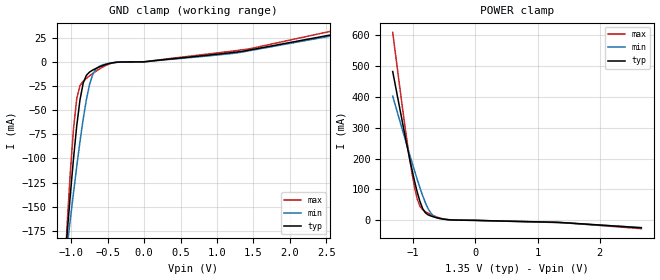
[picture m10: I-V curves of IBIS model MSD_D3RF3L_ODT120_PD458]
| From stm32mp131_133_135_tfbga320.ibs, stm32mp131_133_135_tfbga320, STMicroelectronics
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[Model] MSD_D3RF3L_ODT120_PD458
Model_type   Input
C_comp 2.350pF   2.272pF   2.440pF
Vinh = 810.000mV
Vinl = 540.000mV
[Receiver Thresholds]
Vth   =  0.675V
Vth_min  =  0.6615V
Vth_max  =  0.6885V
Vinh_ac  =  0.160V
Vinh_dc  =  0.090V
Vinl_ac  = -0.160V
Vinl_dc  = -0.090V
Tslew_ac =  5.000ns |Not specified, so set to high value
[Temperature Range]   25.000   125.000   -40.000
[Voltage Range]   1.350V   1.283V   1.450V
[GND Clamp Reference]   0.00V   0.00V   0.00V
[POWER Clamp Reference]   1.350V   1.283V   1.450V
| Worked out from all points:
|   GND clamp passes 1 mA (typ) near -0.43 V on its own axis
|   POWER clamp passes 1 mA (typ) near -0.32 V on its own axis
[GND Clamp]
-1.318V   -446.4mA   -371.4mA   -564.9mA
-1.098V   -221.3mA   -221.2mA   -229.7mA
-1.055V   -178.6mA   -191.9mA   -169mA
-1.011V   -137.8mA   -163.3mA   -114.4mA
-966.7mV  -99.79mA   -135.3mA   -69.1mA
-922.7mV  -66.28mA   -108.3mA   -38.22mA
-834.9mV  -22.17mA   -59.48mA   -20.04mA
-747mV    -10.58mA   -23.42mA   -14.51mA
-659.1mV  -6.847mA   -7.337mA   -9.707mA
-483.3mV  -1.839mA   -1.559mA   -2.399mA
1.45V     12.26mA    11.56mA    13.54mA
2.68V     29.53mA    28.4mA     33.61mA
[Power Clamp]
-1.33V    481.4mA    401.8mA    608.1mA
-1.155V   297.6mA    279.3mA    336.2mA
-1.023V   166.5mA    189.5mA    156.2mA
-978.8mV  126.8mA    160.4mA    107mA
-934.9mV  90.92mA    132mA      68.16mA
-890.9mV  60.38mA    104.8mA    44.96mA
-847mV    37.48mA    79.2mA     34.07mA
-803mV    24.12mA    56.22mA    27.98mA
-715.1mV  14.07mA    22.82mA    18.79mA
-539.4mV  4.851mA    4.565mA    5.806mA
1.438V    -7.703mA   -8.249mA   -7.847mA
2.668V    -24.09mA   -23.31mA   -26.85mA
